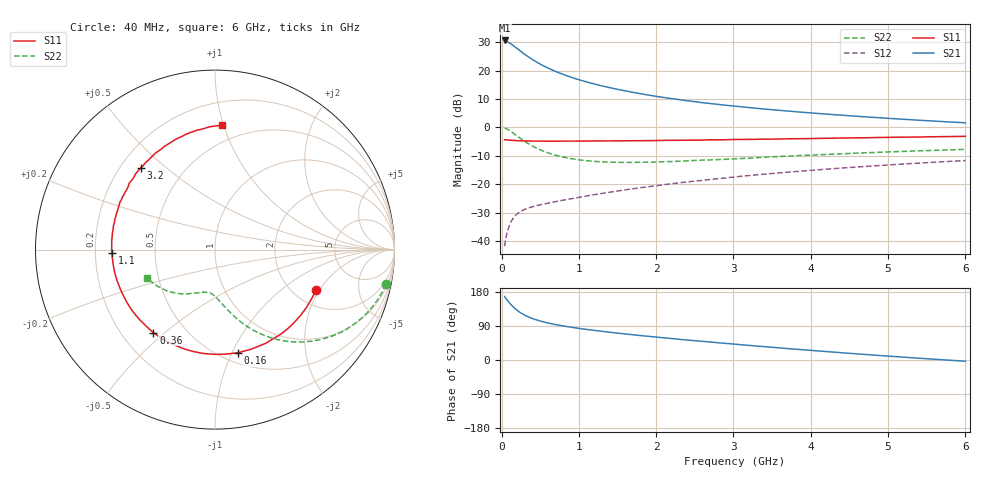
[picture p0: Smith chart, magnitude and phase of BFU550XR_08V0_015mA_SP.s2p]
! Filename:  P:\Prog\Test\Noise\ATS_data\Testdata_Net\03 Spar\BFU550XR_APG2013_45_C05_08p0V_015mA_SP_CM01_D.s2p
! Date/Time: Tue 06/Aug/2013 14:38:17
! BFU550XR_APG2013_45_C05_08p0V_1to35mA_SP_CM01_Bias6_R.s2p
! MDIF S-parameter v. bias file
! BFU550XR_APG2013_45_C05_08p0V_1to35mA_SP_CM01
! Date/time Fri Aug 02 14:53:20 2013
! VAR V_out= 8.0020
! VAR I_out= 15.0000
! VAR V_in= 0.8122
! VAR I_in= 0.1593
! Device data file deembeded for feedlines and parallel
! Original file: \03 Spar\BFU550XR_APG2013_45_C05_08p0V_015mA_SP_CM01_R.s2p
! Feed-files: PR006V01_02082013_Feed1.s2p, PR006V01_02082013_Feed2.s2p
! Parallel-file: PR006V01_02082013_Par.s2p
# MHz S MA R 50
!  Freq-MHz  S11-mag  S11-arg  S21-mag  S21-arg  S12-mag  S12-arg  S22-mag  S22-arg
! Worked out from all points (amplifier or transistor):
!   98 points, 40 MHz to 6 GHz, reference 50 ohm
!   highest |S21| = 30.6 dB at 40 MHz (marker M1)
!   |S21| within 3 dB of that: start of sweep to 209.2 MHz
!   unconditionally stable (mu >= 1): 1.724 GHz to 3.65 GHz
!   at 300 MHz: K = 0.36, MSG = 27.3 dB, |S12| = -28.9 dB
!   at 1.6 GHz: K = 0.98, MSG = 17.4 dB, |S12| = -22.0 dB
!   at 6 GHz: K = 0.88, MSG = 6.7 dB, |S12| = -11.7 dB
!   S11 on the Smith chart (normalised r, x): 40 MHz: 2.60, -1.87; 160 MHz: 0.60, -1.05; 360 MHz: 0.33, -0.46; 1.1 GHz: 0.27, -0.01; 3.2 GHz: 0.28, +0.41; 6 GHz: 0.37, +0.99
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40  0.6065 -22.0  33.93 167.6  0.008091 80.8  0.9691 -11.4
50  0.6039 -27.4  33.64 164.2  0.01 78.9  0.961 -14.3
80  0.5996 -43.0  31.99 156.6  0.01531 72.3  0.9187 -22.5
100  0.5965 -52.7  30.86 151.6  0.01849 68.5  0.8853 -27.4
120  0.5936 -61.8  29.67 146.8  0.02132 65.0  0.8509 -32.0
160  0.5886 -77.6  27.02 138.6  0.02608 59.4  0.7779 -40.0
200  0.5835 -91.2  24.53 131.6  0.02973 55.1  0.7073 -46.7
260  0.5791 -107.3  21.26 123.0  0.03382 50.7  0.6176 -54.6
300  0.5773 -116.2  19.39 118.3  0.03595 48.6  0.567 -58.8
360  0.5755 -126.6  16.99 112.7  0.03852 46.7  0.5046 -64.0
460  0.573 -139.8  13.97 105.3  0.04207 45.3  0.4271 -70.4
600  0.5714 -152.8  11.12 97.7  0.04626 45.3  0.3558 -76.8
800  0.5729 -165.2  8.545 89.8  0.05232 46.7  0.2999 -83.3
1050  0.5745 -176.3  6.602 82.1  0.0602 49.0  0.2635 -89.2
1100  0.5741 -178.2  6.311 80.8  0.06186 49.4  0.2592 -90.3
1500  0.5791 169.2  4.676 71.0  0.07577 51.6  0.2427 -97.6
2050  0.5875 155.9  3.439 59.5  0.0958 52.4  0.2471 -106.0
3100  0.6135 134.2  2.305 40.3  0.1377 50.0  0.283 -120.0
3200  0.6143 132.2  2.234 38.6  0.1418 49.6  0.2872 -121.1
4100  0.6395 116.5  1.756 23.8  0.1793 44.5  0.329 -132.9
5200  0.6725 98.6  1.389 7.4  0.2267 36.5  0.3774 -146.9
6000  0.6953 86.7  1.203 -3.3  0.2599 30.0  0.41 -157.1
